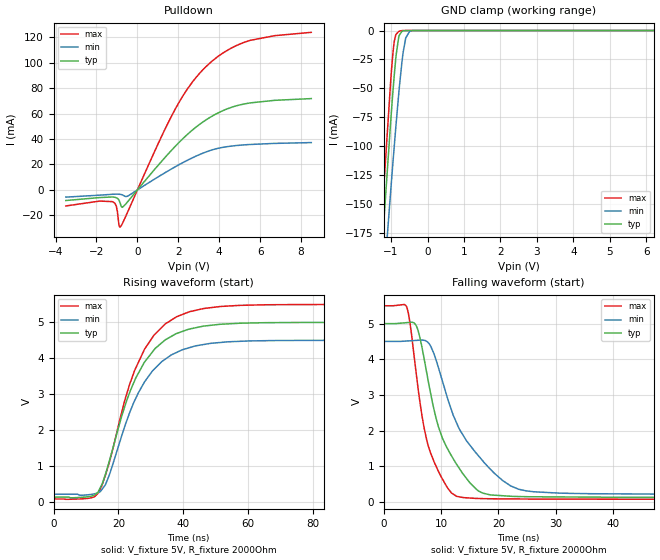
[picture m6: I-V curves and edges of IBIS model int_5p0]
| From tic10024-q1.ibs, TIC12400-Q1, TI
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|   int_5p0 Model
[Model]   int_5p0
Model_type   Open_drain
Polarity   Inverting
Vmeas = 2.5
Vref = 5.0
Cref = 2pF
Rref = 2000
|   typ   min   max
C_comp   3.88723E-12F   3.83388E-12F   3.92321E-12F
| Where nom  PVT is Nominal Process, 5.0V, 27C
|   Fast PVT is Strong Process,  5.5V, -40C
|   Slow PVT is Weak Process,   4.5V, 150C
[Voltage Range]   5   4.5   5.5
|Junction Temperature
[Temperature Range]   27   150   -40
[Pullup Reference]   5   4.5   5.5
[Pulldown Reference]   -0   -0   0
[Power Clamp Reference]   5   4.5   5.5
[GND Clamp Reference]   0   0   0
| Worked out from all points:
|   slope of the pulldown table from 0 to 0.75 V, typ, clamps not added: 52.1 ohm
|   GND clamp passes 1 mA (typ) near -0.71 V on its own axis
|   falling waveform, V_fixture 5V, R_fixture 2000Ohm: 20-80 % time 5.5ns typ, 7.96ns min, 3.64ns max; typ from 5 V to 0.125 V
|   rising waveform, V_fixture 5V, R_fixture 2000Ohm: 20-80 % time 12.1ns typ, 12.1ns min, 11.9ns max; typ from 0.125 V to 5 V
[Pulldown]
|   Voltage   I(typ)   I(min)   I(max)
-3.5V     -8.294mA   -5.581mA   -12.63mA
-1.22V    -5.525mA   -3.404mA   -9.179mA
-1.028V   -6.166mA   -3.32mA    -12.99mA
-896mV    -8.2mA     -3.384mA   -27.86mA
-848mV    -10.11mA   -3.46mA    -29.19mA
-740mV    -13.64mA   -3.858mA   -26.63mA
-572mV    -11.13mA   -5.25mA    -20.77mA
1.696V    31.63mA    16.77mA    58.86mA
2.416V    43.19mA    23.07mA    78.59mA
3.208V    53.44mA    28.91mA    94.5mA
5.224V    67.53mA    35.39mA    115.9mA
8.5V      71.74mA    37.19mA    123.8mA
[GND Clamp]
|   Voltage   I(typ)   I(min)   I(max)
-3.5V     -1.252A    -1.193A    -1.294A
-1.268V   -198.2mA   -246.6mA   -169.3mA
-1.256V   -192.4mA   -241.5mA   -163.1mA
-1.004V   -76.46mA   -136.7mA   -41.39mA
-956mV    -56.27mA   -117.5mA   -22.54mA
-908mV    -37.52mA   -98.7mA    -9.011mA
-872mV    -25mA      -84.94mA   -4.041mA
-776mV    -4.271mA   -50.45mA   -640.5uA
-680mV    -463.2uA   -21.8mA    -22.11uA
-596mV    -37.46uA   -6.351mA   -522.9nA
-440mV    -85.16nA   -223uA     0A
8.5V      0A         0A         0A
[POWER Clamp]
|   Voltage   I(typ)   I(min)   I(max)
-3.5V     0A         0A         0A
0V        0A         0A         0A
8.5V      0A         0A         0A
[Ramp]
R_load = 2000
|   typ   min   max
dV/dt_r   2.92473/1.20752e-08   2.57518/1.20949e-08   3.25528/1.18639e-08
dV/dt_f   2.92473/5.49711e-09   2.57517/7.95934e-09   3.25528/3.634e-09
[Falling Waveform]
V_fixture = 5V
V_fixture_min = 4.5V
V_fixture_max = 5.5V
R_fixture = 2000Ohm
C_fixture = 0F
|   Time   V(typ)   V(min)   V(max)
0s        5V         4.5V       5.5V
3.977ns   5.026V     4.512V     5.475V
5.612ns   4.96V      4.529V     3.673V
7.041ns   4.017V     4.531V     2.074V
8.152ns   3.063V     4.374V     1.38V
10.24ns   1.784V     3.384V     641.7mV
13.88ns   774.1mV    1.859V     123.1mV
20.77ns   174.9mV    596.3mV    87.78mV
26.08ns   146.2mV    286.9mV    81.89mV
200ns     125.5mV    208mV      74.53mV
[Rising Waveform]
V_fixture = 5V
V_fixture_min = 4.5V
V_fixture_max = 5.5V
R_fixture = 2000Ohm
C_fixture = 0F
|   Time   V(typ)   V(min)   V(max)
0s        125.5mV    208mV      74.53mV
10.46ns   135.7mV    190.2mV    91.58mV
13.88ns   296.4mV    259.1mV    249.5mV
17.16ns   1.124V     737.3mV    1.091V
22.41ns   2.787V     2.222V     2.963V
28.03ns   3.894V     3.341V     4.252V
34.46ns   4.516V     3.978V     4.96V
41.88ns   4.816V     4.296V     5.298V
68.1ns    4.994V     4.494V     5.494V
200ns     5V         4.5V       5.5V
